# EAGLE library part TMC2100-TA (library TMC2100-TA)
Standalone Step/Dir driver for two-phase bipolar stepper motor, TQFP48-EP(7x7)
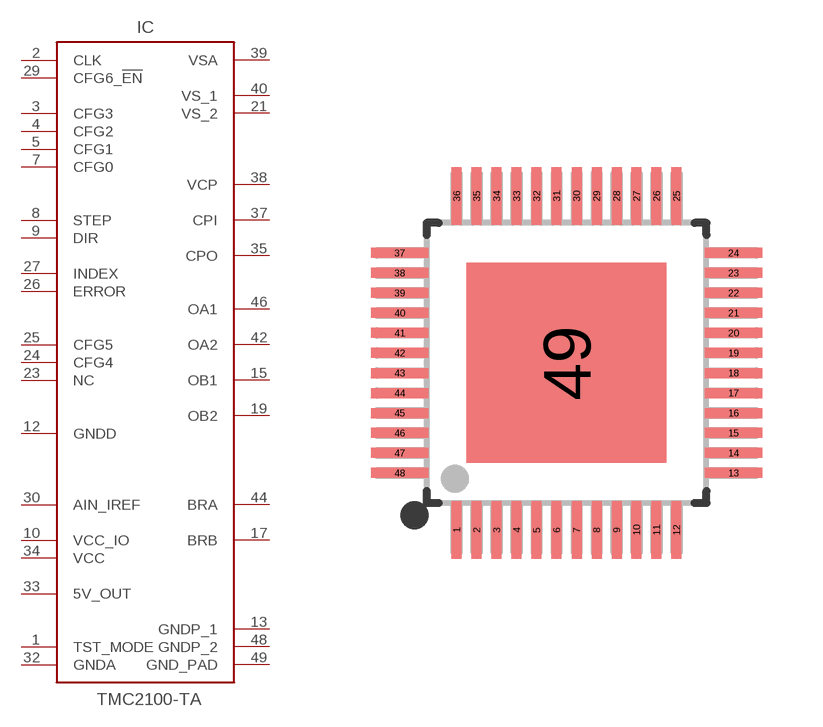
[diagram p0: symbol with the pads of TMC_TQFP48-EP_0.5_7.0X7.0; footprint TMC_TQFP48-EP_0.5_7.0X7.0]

Designator prefix IC

## TMC2100-TA (DATASHEET: http://www.trinamic.com/fileadmin/assets/Products/ICs_Documents/TMC2100_datasheet__1_.pdf; DESCRIPTION: Standalone Step/Dir driver for two-phase bipolar stepper motor, TQFP48-EP(7x7); GEOMETRY_HEIGHT: 1,2mm; MANUFACTURER: TRINAMIC; ORDERCODE-MANU1: TMC2100-TA; VALUE: TMC2100-TA)  [TMC_TQFP48-EP_0.5_7.0X7.0]
1  TST_MODE  in
2  CLK  in
3  CFG3  in
4  CFG2  in
5  CFG1  in
7  CFG0  in
8  STEP  in
9  DIR  in
10  VCC_IO  pwr
12  GNDD  pwr
13  GNDP_1  pwr
15  OB1  out
17  BRB  out
19  OB2  out
21  VS_2  pwr
23  NC  pas
24  CFG4  in
25  CFG5  in
26  ERROR  oc
27  INDEX  oc
29  CFG6_!EN!  in
30  AIN_IREF  in
32  GNDA  pwr
33  5V_OUT  pwr
34  VCC  pwr
35  CPO  out
37  CPI  in
38  VCP  pwr
39  VSA  pwr
40  VS_1  pwr
42  OA2  out
44  BRA  out
46  OA1  out
48  GNDP_2  pwr
49  GND_PAD  pwr

## Footprint TMC_TQFP48-EP_0.5_7.0X7.0 (pad centres in mm)
smd 0.25 x 1.45: 1 -2.75,-4.175; 2 -2.25,-4.175; 3 -1.75,-4.175; 4 -1.25,-4.175; 5 -0.75,-4.175; 6 -0.25,-4.175; 7 0.25,-4.175; 8 0.75,-4.175; 9 1.25,-4.175; 10 1.75,-4.175; 11 2.25,-4.175; 12 2.75,-4.175; 25 2.75,4.175; 26 2.25,4.175; 27 1.75,4.175; 28 1.25,4.175; 29 0.75,4.175; 30 0.25,4.175; 31 -0.25,4.175; 32 -0.75,4.175; 33 -1.25,4.175; 34 -1.75,4.175; 35 -2.25,4.175; 36 -2.75,4.175
smd 1.45 x 0.25: 13 4.175,-2.75; 14 4.175,-2.25; 15 4.175,-1.75; 16 4.175,-1.25; 17 4.175,-0.75; 18 4.175,-0.25; 19 4.175,0.25; 20 4.175,0.75; 21 4.175,1.25; 22 4.175,1.75; 23 4.175,2.25; 24 4.175,2.75; 37 -4.175,2.75; 38 -4.175,2.25; 39 -4.175,1.75; 40 -4.175,1.25; 41 -4.175,0.75; 42 -4.175,0.25; 43 -4.175,-0.25; 44 -4.175,-0.75; 45 -4.175,-1.25; 46 -4.175,-1.75; 47 -4.175,-2.25; 48 -4.175,-2.75
smd 5 x 5: 49 0,0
